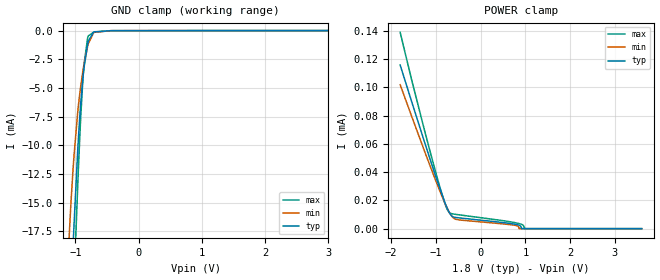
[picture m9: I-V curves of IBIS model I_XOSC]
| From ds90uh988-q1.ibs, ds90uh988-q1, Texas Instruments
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[Model]   I_XOSC
Model_type   Input
Vinl = 0.63
Vinh = 1.17
|   typ   min   max
C_comp   0.878pF   0.919pF   0.838pF
[Voltage Range]   1.8   1.71   1.89
[Temperature Range]   27   105   -40
[Power Clamp Reference]   1.8   1.71   1.89
[GND Clamp Reference]   0   0   0
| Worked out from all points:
|   GND clamp passes 1 mA (typ) near -0.80 V on its own axis
[GND Clamp]
|   Voltage   I(typ)   I(min)   I(max)
-1.8V     -134.8mA   -110.6mA   -157.7mA
-1.147V   -33.59mA   -22.87mA   -42.31mA
-1.071V   -23.15mA   -15.04mA   -29.79mA
-1.028V   -17.62mA   -11.32mA   -22.94mA
-1.022V   -16.96mA   -10.91mA   -22.1mA
-963mV    -10.37mA   -7.066mA   -13.41mA
-930.6mV  -7.442mA   -5.47mA    -9.225mA
-882mV    -4.133mA   -3.537mA   -4.238mA
-865.8mV  -3.3mA     -2.987mA   -3.029mA
-806.4mV  -1.164mA   -1.353mA   -626.1uA
-714.6mV  -140.6uA   -210.9uA   -145.1uA
3.6V      0A         0A         0A
[POWER Clamp]
|   Voltage   I(typ)   I(min)   I(max)
-1.8V     115.8uA    101.8uA    138.9uA
-1.541V   89.65uA    79.31uA    105uA
-979.2mV  34.55uA    31.93uA    36.89uA
-801mV    18.57uA    18.16uA    17.93uA
-698.4mV  11.18uA    11.41uA    11.3uA
-558mV    7.906uA    6.645uA    10.11uA
727.2mV   3.337uA    2.543uA    4.48uA
829.8mV   2.716uA    1.786uA    3.825uA
862.2mV   2.404uA    23.83nA    3.574uA
916.2mV   103.9nA    0A         3.024uA
991.8mV   0A         0A         0A
3.6V      0A         0A         0A
